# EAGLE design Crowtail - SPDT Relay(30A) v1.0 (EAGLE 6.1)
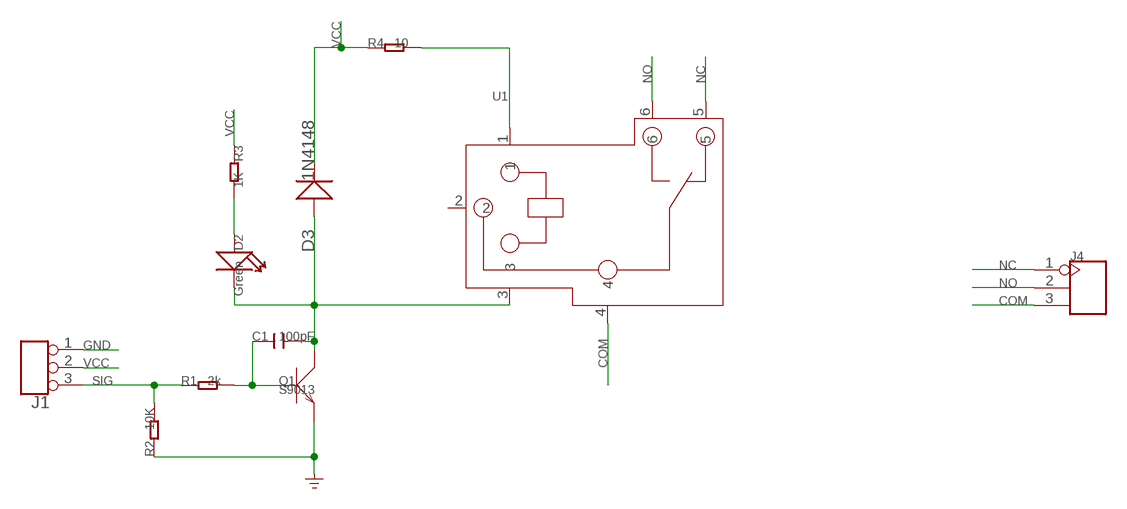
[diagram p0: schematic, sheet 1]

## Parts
C1  100pF  C-0603  [C0603]
D2  Green  LED'0603'  [LED-0603]
D3  1N4148  D'1N4148-SMD'  [DO-35-SMD]
J1  TINKER_3P_DIP  [3P_2.0_DIP]
J4  SCREW-TERMINAL-3P'5.08'  [3P-5.08]
Q1  S9013  TRANSISTOR-NPN-SOT23  [SOT23]
R1  2k  R-0603  [R0603]
R2  10K  R-0603  [R0603]
R3  1K  R-0603  [R0603]
R4  10  R-0603  [R0603]
U1  RELAY-SLA-05VDC-SL-C  [6P-19.8H]

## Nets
COM: J4.3 U1.4
GND: J1.1 Q1.2(E) R2.1
N$1: C1.1 Q1.1(B) R1.2
N$2: D2.+ R3.2
N$3: C1.2 D2.- D3.A(+) Q1.3(C) U1.3
N$7: R4.2 U1.1
NC: J4.1 U1.5
NO: J4.2 U1.6
SIG: J1.3 R1.1 R2.2
VCC: D3.C(-) J1.2 R3.1 R4.1
Unconnected: U1.2

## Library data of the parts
C1 = Discrete:C*: Ceramic Capacitors
D2 = Discrete:LED*
D3 = Discrete:D*
J1 = Connector:TINKER_3P_DIP
J4 = Connector:SCREW-TERMINAL-3P
Q1 = Discrete:TRANSISTOR-NPN*: NPN audion
R1-R4 = Discrete:R*
U1 = template:RELAY-SLA-05VDC-SL-C: · Up to 30A switching in SPST and 20A switching in spot arrangements. · Available as an open-frame relay, with a snap-on dust cover or with an immersion cleanable, plastic sealed case.

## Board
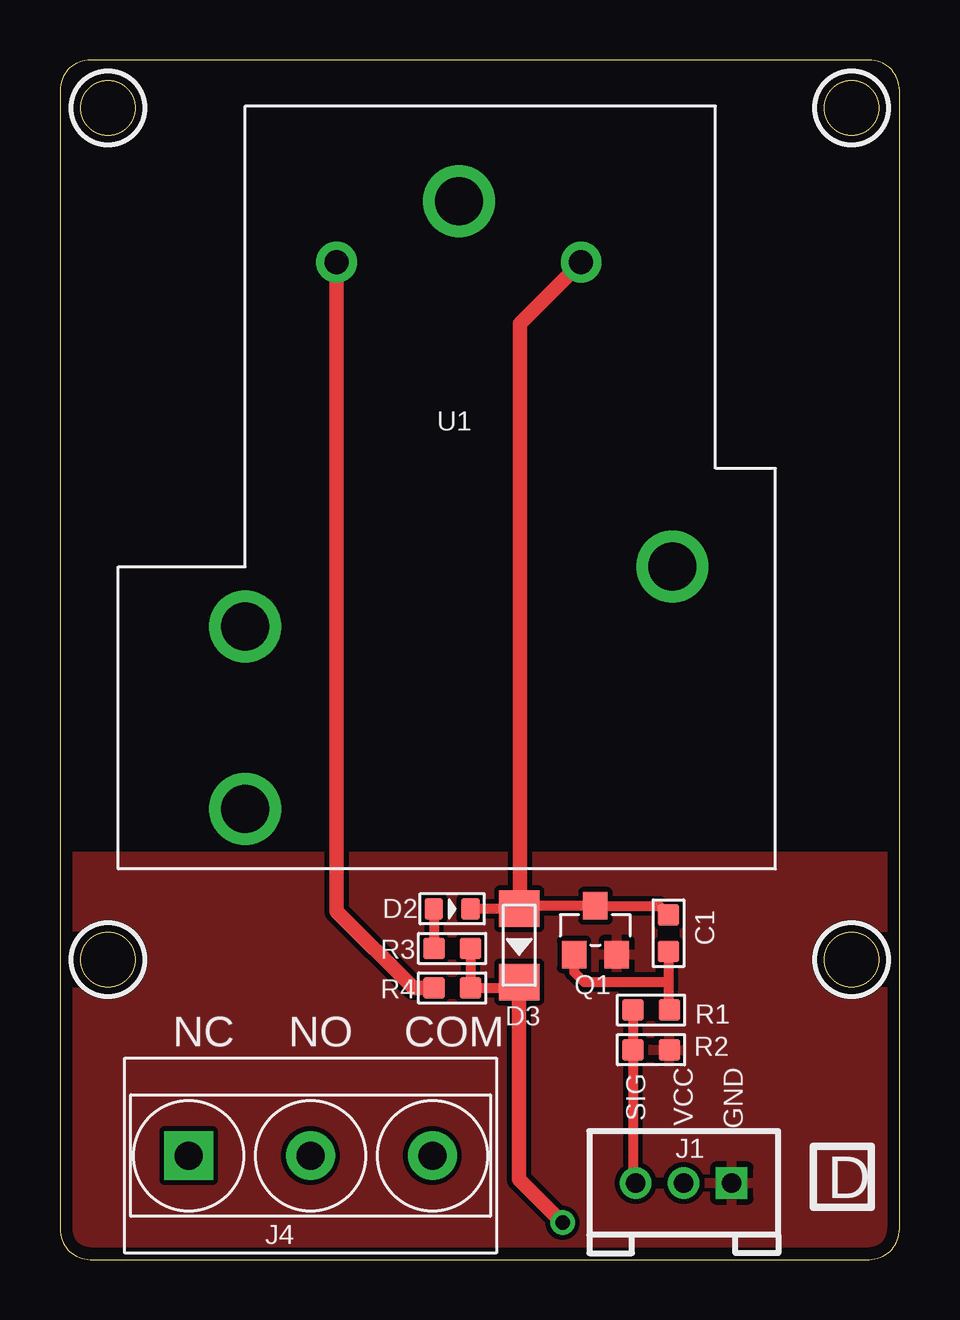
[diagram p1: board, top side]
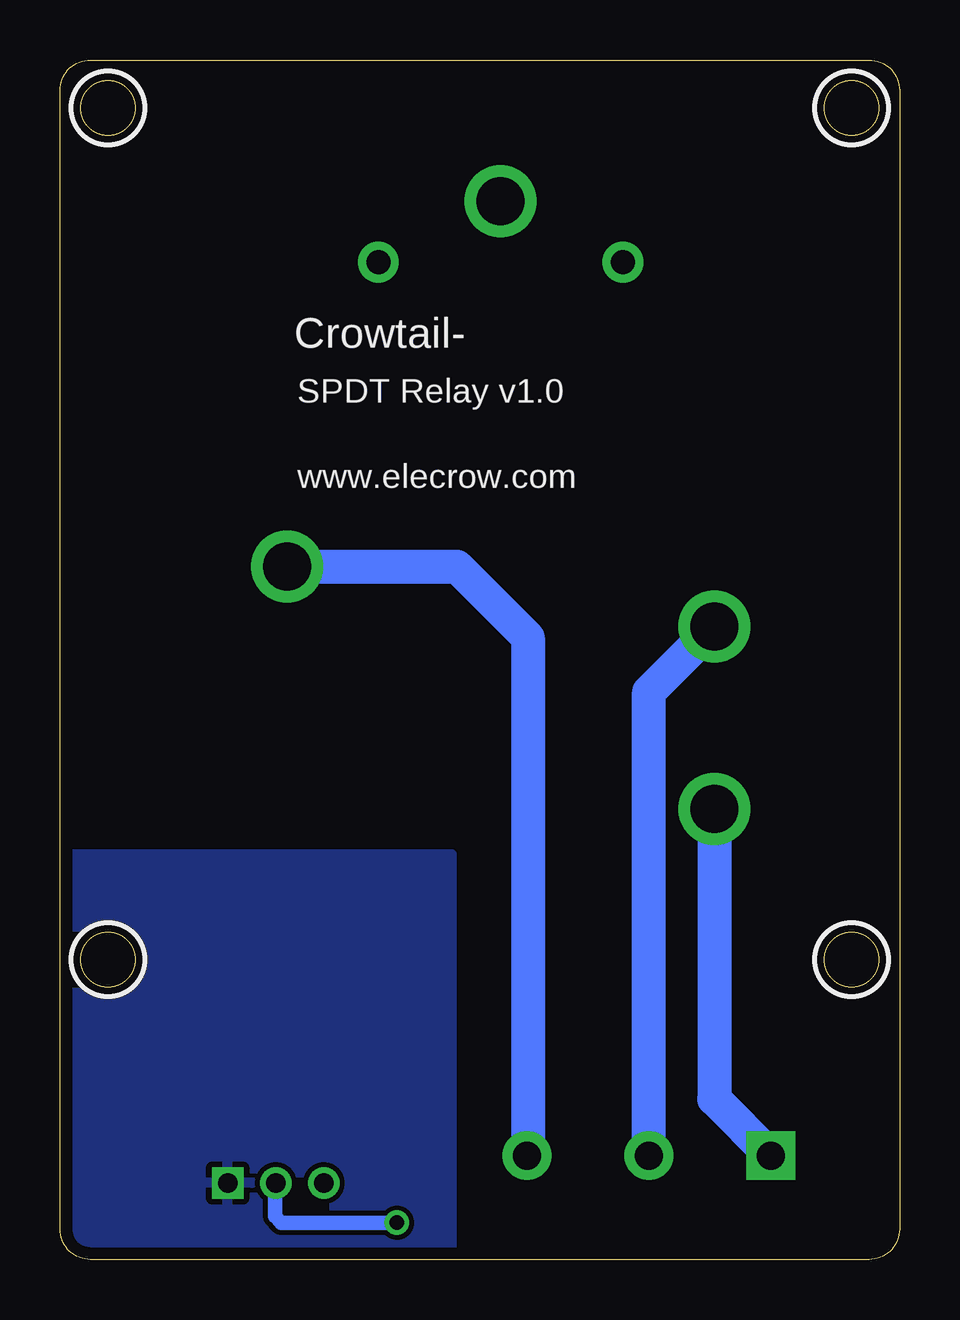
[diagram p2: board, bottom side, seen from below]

Size 35 x 50 mm. Coordinates in mm from the lower left corner, seen from the top.
Outline: 1.27,0 33.73,0 arc90 35,1.27 35,48.73 arc90 33.73,50 1.27,50 arc90 0,48.73 0,1.27 arc90 1.27,0
Outline: circle at 2,48 radius 1.14
Outline: circle at 33,48 radius 1.14
Outline: circle at 2,12.5 radius 1.14
Outline: circle at 33,12.5 radius 1.14
Copper layers (1*16): Top 0.035mm / dielectric 1.5mm / Bottom 0.035mm
Design rules: minimum track width 10mil, minimum drill 12mil, track to track 8mil, track to pad 8mil, pad to pad 8mil, via to via 8mil, smd to smd 0mil, copper to edge 20mil, drill to drill 8mil, minimum pad ring 10mil, minimum via ring 8mil, stop-mask expansion 4mil, vias tented up to drill 100mil, thermal gap 10mil
tRestrict: area 0.5,46.5 to 3.5,49.5; area 31.5,46.5 to 34.5,49.5; area 0.5,11 to 3.5,14; area 31.5,11 to 34.5,14
bRestrict: area 0.5,46.5 to 3.5,49.5; area 31.5,46.5 to 34.5,49.5; area 0.5,11 to 3.5,14; area 31.5,11 to 34.5,14

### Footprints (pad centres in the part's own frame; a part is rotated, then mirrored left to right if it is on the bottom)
C0603 = smd 0.889 x 0.889: 1 -0.762,0; 2 0.762,0
LED-0603 = smd 0.762 x 0.889: + -0.762,0; - 0.762,0
DO-35-SMD = smd 1.524 x 1.676: A -1.524,0; C 1.524,0
3P_2.0_DIP = drill 0.8 pad 1.27 square: 1 -2,0 | drill 0.8 pad 1.27: 2 0,0; 3 2,0
3P-5.08 = drill 1.168 pad 2.032 square: 1 0,5.08 | drill 1.168 pad 2.032: 2 0,0; 3 0,-5.08
SOT23 = smd 1.016 x 1.143: 1 -0.889,-1.016; 2 0.889,-1.016; 3 0,1.016
R0603 = smd 0.889 x 0.889: 1 -0.762,0; 2 0.762,0
6P-19.8H = drill 1 pad 1.7: 1 -9.4,-4.6; 3 -9.4,5.6 | drill 2 pad 3: 2 -11.94,0.5; 4 3.3,9.4; 5 13.4,-8.4; 6 5.8,-8.4

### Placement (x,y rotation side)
C1  25.37,13.6 90 top
D2  16.35,14.62 0 top
D3  19.14,13.1 270 top
J1  26,3.19 180 top
J4  10.45,4.33 90 top
Q1  22.32,13.73 0 top
R1  24.64,10.4 0 top
R2  24.64,8.75 180 top
R3  16.35,12.97 180 top
R4  16.35,11.32 180 top
U1  16.13,32.18 270 top

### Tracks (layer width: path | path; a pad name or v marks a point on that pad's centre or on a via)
COM
  Bottom 1.422: U1.4 18.45,28.88 15.49,25.92 15.49,4.36 J4.3
GND
  pour Bottom: 18.67,-0.24 35.18,-0.24 35.18,16.91 18.67,16.91
  pour Top: -0.13,-0.24 35.31,-0.24 35.31,16.78 -0.13,16.78
N$1
  Top 0.406: C1.1 25.37,11.44 | 25.37,11.44 25.37,10.43 R1.2 | Q1.1 21.43,11.98 21.84,11.57 25.24,11.57 25.37,11.44
N$2
  Top 0.406: D2.+ R3.2
N$3
  Top 0.406: D2.- D3.A 19.27,14.75 Q1.3 24.99,14.75 C1.2
  Top 0.61: U1.3 21.73,41.55 19.18,39 19.18,14.65 D3.A
N$7
  Top 0.61: U1.1 11.53,14.52 14.73,11.32 R4.2
NC
  Bottom 1.422: U1.5 7.73,6.7 J4.1
NO
  Bottom 1.422: J4.2 10.45,23.66 U1.6
SIG
  Top 0.406: R1.1 R2.2 23.88,3.32 J1.3
VCC  (via drill 0.61)
  Top 0.406: R3.1 R4.1 18.89,11.32 D3.C
  Top 0.61: D3.C 19.14,3.35 v20.95,1.54
  Bottom 0.61: v20.95,1.54 25.78,1.54 26.04,1.79 26.04,3.16 J1.2

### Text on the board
tPlace: NC | NO | COM | SIG | VCC | GND | D
bPlace: Crowtail- | SPDT Relay v1.0 | www.elecrow.com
